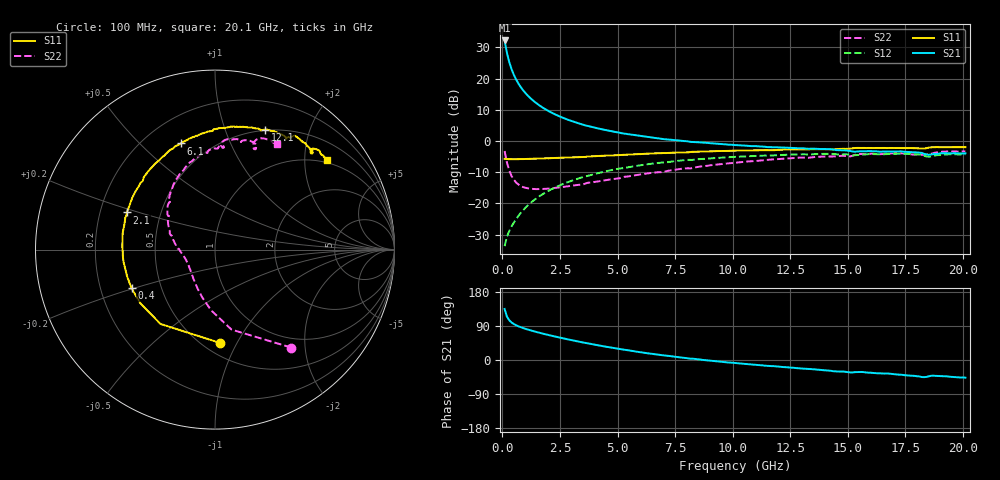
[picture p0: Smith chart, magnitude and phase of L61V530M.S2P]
!  Infineon Technologies AG
! BFR380L3 , PF131585-7, No.6, Th 09.10.01, soldered on pcb-board, measured with PP GSG850
!  Vce=1.5 V,  Ic=30.0 mA
! Common Emitter S-Parameters:  15. November 2001
#  GHz  S  MA  R  50
! f  S11  S21  S12  S22
! GHz  Mag  Ang  Mag  Ang  Mag  Ang  Mag  Ang
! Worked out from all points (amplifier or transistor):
!   201 points, 100 MHz to 20.1 GHz, reference 50 ohm
!   highest |S21| = 32.2 dB at 100 MHz (marker M1)
!   |S21| within 3 dB of that: start of sweep to 176.4 MHz
!   unconditionally stable (mu >= 1): 1.122 GHz to 4.461 GHz
!   at 3.4 GHz: K = 1.02, MAG = 7.8 dB, |S12| = -11.8 dB
!   at 10.1 GHz: K = 0.97, MSG = 1.9 dB, |S12| = -5.1 dB
!   at 20.1 GHz: K = 0.99, MSG = 0.2 dB, |S12| = -4.2 dB
!   S11 on the Smith chart (normalised r, x): 100 MHz: 0.60, -0.85; 400 MHz: 0.34, -0.20; 2.1 GHz: 0.32, +0.18; 6.1 GHz: 0.35, +0.67; 12.1 GHz: 0.49, +1.39; 20.1 GHz: 0.93, +2.56
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0.1  0.5196 -87.2  40.81 134.6  0.02073 60.3  0.6912 -52.1
0.2  0.5135 -126.2  25.97 114.5  0.02933 55.0  0.4552 -78.3
0.3  0.5122 -144.2  18.47 105.0  0.03602 56.4  0.339 -93.7
0.4  0.5124 -155.1  14.21 99.1  0.04278 59.1  0.2763 -104.8
0.5  0.5121 -162.6  11.51 94.9  0.04938 61.5  0.2398 -113.5
0.6  0.5114 -167.7  9.658 91.7  0.05629 63.1  0.2168 -120.6
0.7  0.5141 -172.1  8.327 88.9  0.06344 64.4  0.2015 -126.7
0.8  0.5147 -175.4  7.313 86.5  0.07069 65.4  0.1908 -131.8
0.9  0.5144 -178.7  6.522 84.3  0.07789 66.0  0.1833 -136.2
1.1  0.5175 176.1  5.374 80.4  0.0928 66.5  0.1756 -143.5
1.4  0.5227 169.5  4.255 75.2  0.1151 66.4  0.1703 -151.7
1.7  0.5249 163.9  3.533 70.5  0.1373 65.5  0.1707 -158.1
2.1  0.5326 157.2  2.898 64.6  0.1668 63.6  0.1747 -164.6
2.7  0.5444 147.9  2.301 56.3  0.2097 60.0  0.1857 -173.0
3.5  0.5549 136.8  1.829 46.2  0.2649 54.5  0.2017 178.7
6.1  0.6218 107.9  1.191 19.5  0.415 36.0  0.2957 151.9
6.8  0.6389 101.3  1.101 13.6  0.4484 30.7  0.3176 144.7
10.1  0.7015 77.3  0.862 -7.9  0.558 9.2  0.45 118.1
12.1  0.7246 67.2  0.7891 -17.9  0.5996 -2.5  0.5168 103.1
13.5  0.7394 60.4  0.755 -24.6  0.6159 -10.7  0.5509 93.9
16.8  0.7748 48.1  0.6796 -36.1  0.6204 -26.0  0.6315 74.7
20.1  0.7985 38.5  0.6368 -46.7  0.6144 -39.3  0.6842 59.6
